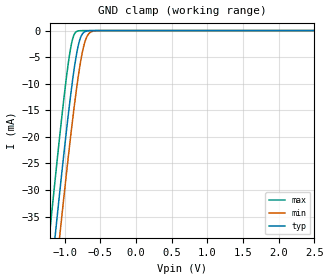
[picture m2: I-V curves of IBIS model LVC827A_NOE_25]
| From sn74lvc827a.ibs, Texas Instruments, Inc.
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[Model]   LVC827A_NOE_25
Model_type  Input
Vinl = 0.7
Vinh = 1.7
| variable   typ   min   max
C_comp   3.96pF   3.14pF   4.73pF
[Temperature Range]   40   100   -40
| Ambient temperature   25   85   -40
[Voltage range]   2.5   2.3   2.7
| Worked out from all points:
|   GND clamp passes 1 mA (typ) near -0.77 V on its own axis
[GND Clamp]
| LVC827A_NOE_25
|   Voltage   I(typ)   I(min)   I(max)
-5V       -584.4mA   -591.4mA   -575.6mA
-1.225V   -50.97mA   -59.27mA   -40.34mA
-1.2V     -47.65mA   -55.95mA   -37mA
-1.13V    -38.46mA   -46.75mA   -27.8mA
-1.07V    -30.74mA   -39mA      -20.15mA
-1.05V    -28.21mA   -36.45mA   -17.67mA
-955mV    -16.69mA   -24.69mA   -6.88mA
-885mV    -9.107mA   -16.56mA   -1.487mA
-780mV    -1.473mA   -6.233mA   -17.16uA
-710mV    -173.9uA   -1.92mA    -639.6nA
-645mV    -18.5uA    -388uA     -30.01nA
2.5V      4.713pA    7.579pA    4.389pA
